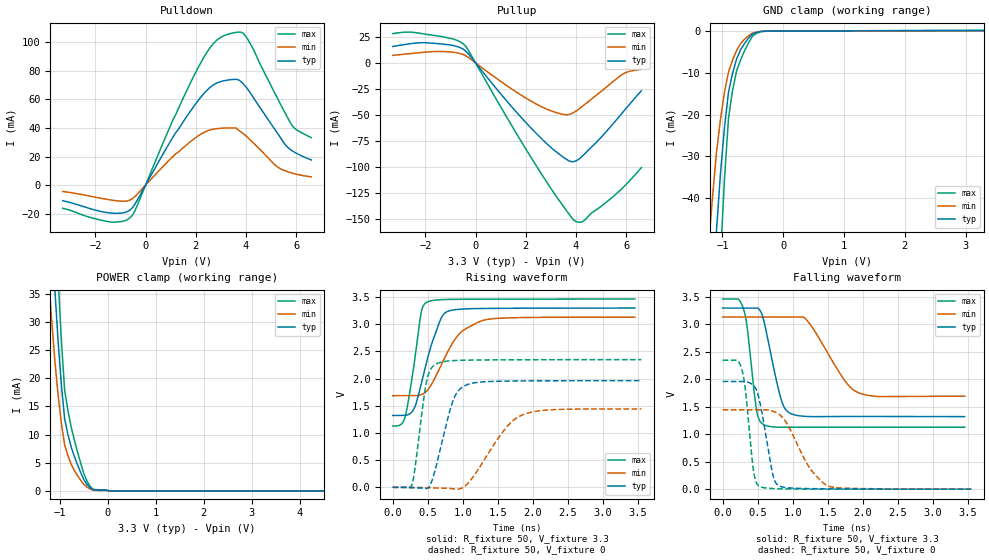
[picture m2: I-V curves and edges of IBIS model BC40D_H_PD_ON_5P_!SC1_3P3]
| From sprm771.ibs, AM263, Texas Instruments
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|   Model Cell BC40D_H_PD_ON_5P_!SC1_3P3
|BC40D_H_PD_ON_5P_!SC1_3P3
[Model]   BC40D_H_PD_ON_5P_!SC1_3P3
Model_type   I/O
Polarity   Non-Inverting
Enable   Active-Low
Vinl =  0.8V
Vinh =  2V
Cref =  15pF
Rref =  100.0000M
Vref =  0V
Vmeas =  1.65
C_comp   2.157014p   1.964007p   2.198404p
|[Input load] weak_pd_on
|[Output drive] fast
|[supplytol] 5
|[temp] ind
[Model Spec]
Vinl   0.8V   0.8V   0.8V
Vinh   2V   2V   2V
[Temperature Range]   25   125   -40
[Voltage Range]   3.3   3.135   3.465
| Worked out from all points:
|   slope of the pulldown table from 0 to 0.495 V, typ, clamps not added: 31.8 ohm
|   slope of the pullup table from 0 to 0.495 V, typ, clamps not added: 33.3 ohm
|   GND clamp passes 1 mA (typ) near -0.52 V on its own axis
|   POWER clamp passes 1 mA (typ) near -0.42 V on its own axis
|   rising waveform, R_fixture 50, V_fixture 3.3: 20-80 % time 258ps typ, 378ps min, 156ps max; typ from 1.32 V to 3.3 V
|   rising waveform, R_fixture 50, V_fixture 0: 20-80 % time 233ps typ, 458ps min, 142ps max; typ from 0 V to 1.96 V
|   falling waveform, R_fixture 50, V_fixture 3.3: 20-80 % time 199ps typ, 411ps min, 121ps max; typ from 3.3 V to 1.32 V
|   falling waveform, R_fixture 50, V_fixture 0: 20-80 % time 162ps typ, 365ps min, 108ps max; typ from 1.96 V to 0 V
| Nom Voltages:
|   VDD=1.1, VDDS=3.3, VDDS18=1.8, ESD_BIASFET=0, VSS=0, VSSS=0
| Min Voltages:
|   VDD=1.045, VDDS=3.135, VDDS18=1.71, ESD_BIASFET=0, VSS=0, VSSS=0
| Max Voltages:
|   VDD=1.16, VDDS=3.465, VDDS18=1.89, ESD_BIASFET=0, VSS=0, VSSS=0
[POWER_clamp]
|   voltage   I(typ)   I(min)   I(max)
-3.3V     446.9mA    437.1mA    604mA
-1.233V   56.59mA    37.52mA    80.37mA
-1.167V   45.68mA    29.91mA    65.17mA
-1.1V     35.14mA    22.67mA    50.36mA
-1.033V   26.13mA    16.78mA    37.31mA
-966.7mV  18.67mA    11.95mA    26.46mA
-900mV    12.76mA    8.173mA    17.82mA
-833.3mV  10.07mA    6.293mA    14.34mA
-566.7mV  3.276mA    1.91mA     4.968mA
-366.7mV  519.9uA    314uA      774.5uA
33.33mV   0A         0A         0A
6.6V      0A         0A         0A
[Pulldown]
|   voltage   I(typ)   I(min)   I(max)
-3.3V     -10.92mA   -4.469mA   -16.24mA
-1.4V     -19.52mA   -10.37mA   -25.81mA
-600mV    -17.22mA   -10.34mA   -22.6mA
-400mV    -12.67mA   -7.623mA   -17.05mA
1.2V      36.7mA     21.92mA    49.35mA
2.1V      59.3mA     34.49mA    82.4mA
2.7V      70.09mA    39.15mA    99.03mA
3.3V      73.56mA    39.95mA    105.7mA
3.9V      70.66mA    35.84mA    106mA
5.2V      37.64mA    13.39mA    62.46mA
5.8V      24.43mA    8.578mA    42.66mA
6.6V      17.6mA     5.765mA    33.17mA
[Pullup]
|   voltage   I(typ)   I(min)   I(max)
-3.3V     15.77mA    7.22mA     28.03mA
-2.7V     18.05mA    8.673mA    29.54mA
-1.9V     19.23mA    10.53mA    27.2mA
-900mV    16.69mA    10.25mA    22.94mA
-400mV    11.53mA    6.969mA    16.15mA
1.4V      -40.96mA   -24.37mA   -58.54mA
2.6V      -72.01mA   -41.71mA   -105.6mA
3.6V      -92.16mA   -49.74mA   -141mA
4V        -93.88mA   -46.2mA    -152.2mA
4.3V      -88.33mA   -40.72mA   -151.7mA
5.9V      -46.29mA   -10.2mA    -118.8mA
6.6V      -26.71mA   -6.269mA   -100.4mA
[GND_clamp]
|   voltage   I(typ)   I(min)   I(max)
-3.3V     -787.2mA   -627.7mA   -1.235A
-1.233V   -85.66mA   -52.14mA   -138.8mA
-1.167V   -66.47mA   -40.37mA   -107.7mA
-1.1V     -48.25mA   -29.37mA   -77.98mA
-1.033V   -34.28mA   -21.19mA   -54.56mA
-966.7mV  -23.07mA   -14.67mA   -35.51mA
-900mV    -14.62mA   -9.792mA   -20.84mA
-833.3mV  -10.07mA   -6.939mA   -14.17mA
-700mV    -4.435mA   -2.94mA    -6.836mA
-500mV    -641.2uA   -454.9uA   -1.12mA
-300mV    -31.62uA   -32.88uA   -44.11uA
3.3V      108.6uA    60.68uA    188uA
[Ramp]
| variable   typ   min   max
dV/dt_f  1.1954796/0.20075621n 0.88994094/0.42402921n  1.4066403/0.12168663n
dV/dt_r  1.1916358/0.23564931n 0.88865982/0.46962037n  1.4192669/0.14321042n
R_load = 50
[Rising Waveform]
R_fixture = 50
V_fixture = 3.3
V_fixture_min = 3.135
V_fixture_max = 3.465
|   time   V(typ)   V(min)   V(max)
0s        1.321V     1.685V     1.128V
177.4ps   1.322V     1.685V     1.297V
303.5ps   1.443V     1.685V     2.248V
401.9ps   1.879V     1.701V     3.185V
484.7ps   2.311V     1.769V     3.403V
665.2ps   3.031V     2.177V     3.449V
735.7ps   3.195V     2.366V     3.453V
958.1ps   3.275V     2.831V     3.458V
1.252ns   3.288V     3.053V     3.46V
3.453ns   3.297V     3.129V     3.462V
[Rising Waveform]
R_fixture = 50
V_fixture = 0
V_fixture_min = 0
V_fixture_max = 0
|   time   V(typ)   V(min)   V(max)
0s        0V         0V         0V
274.9ps   -6.689mV   0V         52.25mV
480.5ps   -23.36mV   -4.905mV   1.934V
543.2ps   65.04mV    -6.663mV   2.176V
622.8ps   403.3mV    -9.009mV   2.269V
861.3ps   1.596V     -28.02mV   2.33V
1.052ns   1.882V     46.58mV    2.339V
1.589ns   1.953V     1.05V      2.345V
1.843ns   1.956V     1.327V     2.346V
3.547ns   1.962V     1.442V     2.348V
[Falling Waveform]
R_fixture = 50
V_fixture = 3.3
V_fixture_min = 3.135
V_fixture_max = 3.465
|   time   V(typ)   V(min)   V(max)
0s        3.298V     3.134V     3.461V
301ps     3.298V     3.134V     3.263V
347.8ps   3.298V     3.134V     2.961V
482.3ps   3.298V     3.134V     1.448V
586.8ps   3.065V     3.134V     1.174V
826.2ps   1.665V     3.134V     1.128V
968.8ps   1.377V     3.134V     1.128V
1.198ns   1.324V     3.079V     1.129V
1.927ns   1.324V     1.762V     1.127V
3.453ns   1.321V     1.694V     1.127V
[Falling Waveform]
R_fixture = 50
V_fixture = 0
V_fixture_min = 0
V_fixture_max = 0
|   time   V(typ)   V(min)   V(max)
0s        1.961V     1.447V     2.348V
273.2ps   1.961V     1.447V     2.18V
322.1ps   1.958V     1.447V     1.829V
437.9ps   1.888V     1.447V     344.1mV
525.3ps   1.61V      1.447V     50.61mV
715ps     262.7mV    1.42V      11.51mV
813.4ps   54.79mV    1.354V     6.577mV
1.252ns   9.379mV    365.9mV    0V
1.507ns   6.075mV    57.24mV    0V
3.547ns   0V         2.907mV    0V
